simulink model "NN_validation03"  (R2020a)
settings: Solver=ode45  StartTime=0.0  StopTime=2000  RelTol=1e-3  EnableMultiTasking=on
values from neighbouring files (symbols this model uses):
  Ts = 0.2    [init_model.m]
libraries: neural x26

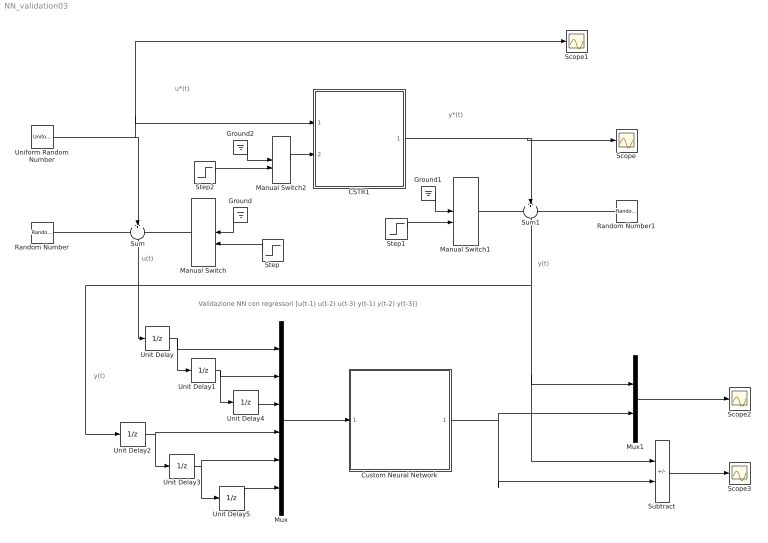
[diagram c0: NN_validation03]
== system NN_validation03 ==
  note: u(t)
  note: u*(t)
  note: y(t)
  note: y*(t)
  note: Validazione NN con regressori [u(t-1) u(t-2) u(t-3) y(t-1) y(t-2) y(t-3)]
  note: y(t)
  CSTR1 : Subsystem
  Custom Neural Network : Subsystem
      mask help: Custom Neural Network
  Ground : Ground
  Ground1 : Ground
  Ground2 : Ground
  Manual Switch : ManualSwitch  CurrentSetting=0
  Manual Switch1 : ManualSwitch
  Manual Switch2 : ManualSwitch
  Mux : Mux  Inputs=6
  Mux1 : Mux  Inputs=2
  Random Number : RandomNumber  Variance=0.0001  Seed=1  SampleTime=Ts
  Random Number1 : RandomNumber  Variance=0.0005  Seed=2  SampleTime=Ts
  Scope{,1..3} (4 alike) : Scope
  Step : Step  Time=1000  After=10  SampleTime=0
  Step1 : Step  Time=1000  After=10  SampleTime=0
  Step2 : Step  Time=1000  SampleTime=0
  Subtract : Sum  Inputs=+-
  Sum : Sum  Inputs=+++  SaturateOnIntegerOverflow=on
  Sum1 : Sum  Inputs=+++  SaturateOnIntegerOverflow=on
  Uniform Random Number : UniformRandomNumber  Minimum=0  Maximum=4  SampleTime=20
  Unit Delay{,1..5} (6 alike) : UnitDelay  SampleTime=Ts  HasFrameUpgradeWarning=on
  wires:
  Uniform Random Number/1 -> CSTR1/1(w), Scope1/1, Sum/2
  Random Number/1 -> Sum/1
  Manual Switch/1 -> Sum/3
  Sum/1 -> Unit Delay/1
  Ground/1 -> Manual Switch/1
  Step/1 -> Manual Switch/2
  Ground1/1 -> Manual Switch1/1
  Step1/1 -> Manual Switch1/2
  CSTR1/1(Cb) -> Scope/1, Sum1/2
  Manual Switch1/1 -> Sum1/1
  Random Number1/1 -> Sum1/3
  Unit Delay/1 -> Mux/1, Unit Delay1/1
  Unit Delay2/1 -> Unit Delay3/1, Mux/4
  Step2/1 -> Manual Switch2/2
  Manual Switch2/1 -> CSTR1/2(f)
  Ground2/1 -> Manual Switch2/1
  Unit Delay1/1 -> Mux/2, Unit Delay4/1
  Unit Delay4/1 -> Mux/3
  Unit Delay5/1 -> Mux/6
  Unit Delay3/1 -> Mux/5, Unit Delay5/1
  Mux/1 -> Custom Neural Network/1(Input)
  Subtract/1 -> Scope3/1
  Mux1/1 -> Scope2/1
  Sum1/1 -> Subtract/1, Mux1/1, Unit Delay2/1
  Custom Neural Network/1(Output) -> Subtract/2, Mux1/2

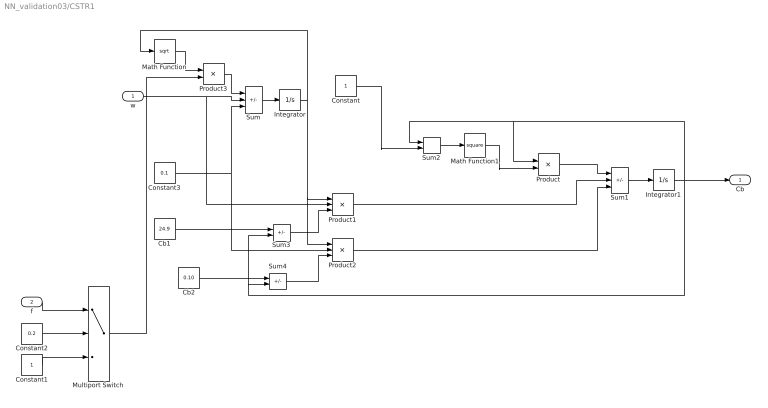
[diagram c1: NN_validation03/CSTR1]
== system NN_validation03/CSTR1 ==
  w : Inport
  f : Inport  Port=2
  Cb1 : Constant  Value=24.9
  Cb2 : Constant  Value=0.10
  Constant : Constant
  Constant1 : Constant
  Constant2 : Constant  Value=0.2
  Constant3 : Constant  Value=0.1
  Integrator : Integrator  InitialCondition=30  LimitOutput=on  LowerSaturationLimit=1
  Integrator1 : Integrator  InitialCondition=22
  Math Function : Math  Operator=sqrt
  Math Function1 : Math  Operator=square
  Multiport Switch : MultiPortSwitch  DataPortOrder=Zero-based contiguous  Inputs=2  zeroidx=on
  Product : Product  Inputs=*/  SaturateOnIntegerOverflow=on
  Product1 : Product  Inputs=/**  SaturateOnIntegerOverflow=on
  Product2 : Product  Inputs=/**  SaturateOnIntegerOverflow=on
  Product3 : Product
  Sum : Sum  Inputs=-++  SaturateOnIntegerOverflow=on
  Sum1 : Sum  Inputs=-++  SaturateOnIntegerOverflow=on
  Sum2 : Sum  SaturateOnIntegerOverflow=on
  Sum3 : Sum  Inputs=+-  SaturateOnIntegerOverflow=on
  Sum4 : Sum  Inputs=+-  SaturateOnIntegerOverflow=on
  Cb : Outport
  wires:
  Sum/1 -> Integrator/1
  Product3/1 -> Sum/1
  Math Function/1 -> Product3/1
  Integrator/1 -> Math Function/1, Product1/1, Product2/1
  Sum3/1 -> Product1/3
  Sum4/1 -> Product2/3
  Sum2/1 -> Math Function1/1
  Sum1/1 -> Integrator1/1
  Math Function1/1 -> Product/2
  Product/1 -> Sum1/1
  Product1/1 -> Sum1/2
  Product2/1 -> Sum1/3
  w/1 -> Sum/2, Product1/2
  Constant3/1 -> Product2/2, Sum/3
  Integrator1/1 -> Sum3/2, Sum4/2, Sum2/1, Product/1, Cb/1
  Constant1/1 -> Multiport Switch/3
  f/1 -> Multiport Switch/1
  Constant2/1 -> Multiport Switch/2
  Cb2/1 -> Sum4/1
  Cb1/1 -> Sum3/1
  Constant/1 -> Sum2/2
  Multiport Switch/1 -> Product3/2

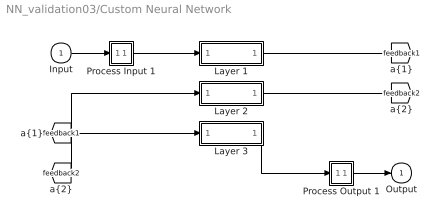
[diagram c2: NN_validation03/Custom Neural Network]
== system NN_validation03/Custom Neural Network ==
  Input : Inport  PortDimensions=6  SampleTime=0.2
  Layer 1 : Subsystem
  Layer 2 : Subsystem
  Layer 3 : Subsystem
  Process Input 1 : Subsystem
  Process Output 1 : Subsystem
  Output : Outport  InitialOutput=0
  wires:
  Input/1 -> Process Input 1/1(x)
  Process Output 1/1(y) -> Output/1
  Process Input 1/1(p) -> Layer 1/1("p{1}")
  Layer 1/1("a{1}") -> [feedback1]
  [feedback1] -> Layer 2/1("a{1} ")
  Layer 2/1("a{2}") -> [feedback2]
  [feedback2] -> Layer 3/1("a{2} ")
  Layer 3/1("a{3}") -> Process Output 1/1(a)

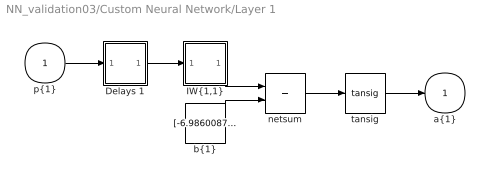
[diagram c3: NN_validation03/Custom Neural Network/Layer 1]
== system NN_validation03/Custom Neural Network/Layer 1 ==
  "p{1}" : Inport  PortDimensions=6  SampleTime=0.2
  Delays 1 : Subsystem
  "IW{1,1}" : Subsystem
  "b{1}" : Constant  Value=[-6.9860087142336624310701154172420501708984375;-1.3825822154357074733610488692647777497768402099609375;1.414744489111007030857081190333701670169830322265625;1.4343419531810190914455915844882838428020477294921875;0.364071132160834254332115733632235787808895111083984375;-0.2427588004599351700907305939836078323423862457275390625;-1.3732031975720901950666075208573602139949798583984375]
  netsum : Sum  Inputs=2  InputSameDT=on  SaturateOnIntegerOverflow=on
  tansig : neural/Transfer Functions/tansig
  "a{1}" : Outport  InitialOutput=[0;0;0;0;0;0;0]
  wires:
  "p{1}"/1 -> Delays 1/1("p{1}")
  Delays 1/1("pd{1,1}") -> "IW{1,1}"/1("pd{1,1}")
  "IW{1,1}"/1("iz{1,1}") -> netsum/1
  "b{1}"/1 -> netsum/2
  netsum/1 -> tansig/1
  tansig/1 -> "a{1}"/1

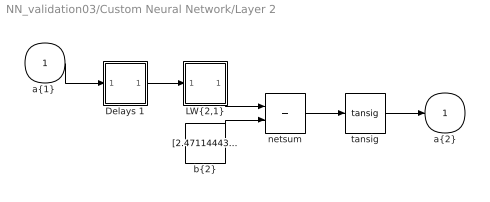
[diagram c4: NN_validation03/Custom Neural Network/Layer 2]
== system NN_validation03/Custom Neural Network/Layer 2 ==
  "a{1} " : Inport  PortDimensions=7  SampleTime=0.2
  Delays 1 : Subsystem
  "LW{2,1}" : Subsystem
  "b{2}" : Constant  Value=[2.471144434973719938852809718810021877288818359375;2.563750047572993739919411382288672029972076416015625;1.6633879212355908716602925778715871274471282958984375;-0.94058786412804240573137803949066437780857086181640625;-0.10710243137428977766578697128352359868586063385009765625;0.10718094125826170548432259010951383970677852630615234375;0.036160654709730725986371879798753070645034313201904296875;-0.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
  netsum : Sum  Inputs=2  InputSameDT=on  SaturateOnIntegerOverflow=on
  tansig : neural/Transfer Functions/tansig
  "a{2}" : Outport  InitialOutput=[0;0;0;0;0;0;0;0;0;0;0;0;0;0;0]
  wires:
  "a{1} "/1 -> Delays 1/1("p{2}")
  Delays 1/1("pd{2,1}") -> "LW{2,1}"/1("ad{2,1}")
  "LW{2,1}"/1("lz{2,1}") -> netsum/1
  "b{2}"/1 -> netsum/2
  netsum/1 -> tansig/1
  tansig/1 -> "a{2}"/1

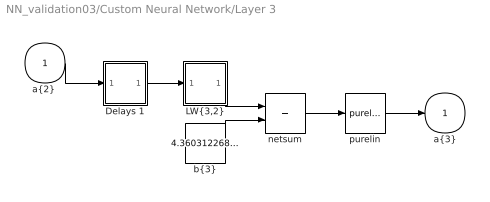
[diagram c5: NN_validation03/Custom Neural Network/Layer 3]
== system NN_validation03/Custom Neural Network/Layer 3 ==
  "a{2} " : Inport  PortDimensions=15  SampleTime=0.2
  Delays 1 : Subsystem
  "LW{3,2}" : Subsystem
  "b{3}" : Constant  Value=4.36031226847928454759539818041957914829254150390625
  netsum : Sum  Inputs=2  InputSameDT=on  SaturateOnIntegerOverflow=on
  purelin : neural/Transfer Functions/purelin
  "a{3}" : Outport  InitialOutput=0
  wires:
  "a{2} "/1 -> Delays 1/1("p{3}")
  Delays 1/1("pd{3,2}") -> "LW{3,2}"/1("ad{3,2}")
  "LW{3,2}"/1("lz{3,2}") -> netsum/1
  "b{3}"/1 -> netsum/2
  netsum/1 -> purelin/1
  purelin/1 -> "a{3}"/1

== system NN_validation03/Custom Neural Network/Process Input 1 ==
  x : Inport  PortDimensions=6  SampleTime=0.2
  p : Outport  PortDimensions=6  SampleTime=0.2
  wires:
  x/1 -> p/1

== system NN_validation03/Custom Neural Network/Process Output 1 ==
  a : Inport  PortDimensions=1  SampleTime=0.2
  y : Outport  PortDimensions=1  SampleTime=0.2
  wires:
  a/1 -> y/1

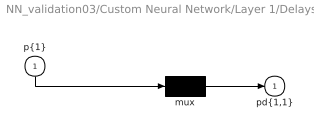
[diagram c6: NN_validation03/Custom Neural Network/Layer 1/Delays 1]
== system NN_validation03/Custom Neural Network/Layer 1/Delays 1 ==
  "p{1}" : Inport  PortDimensions=6  SampleTime=0.2
  mux : Mux  Inputs=1
  "pd{1,1}" : Outport
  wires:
  "p{1}"/1 -> mux/1
  mux/1 -> "pd{1,1}"/1

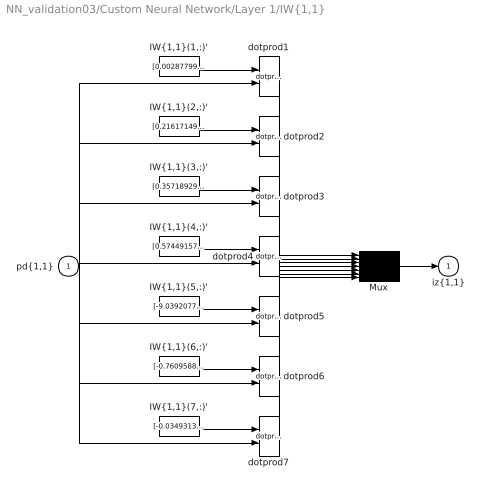
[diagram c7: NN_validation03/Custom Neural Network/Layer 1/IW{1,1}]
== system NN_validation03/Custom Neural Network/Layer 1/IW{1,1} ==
  "pd{1,1}" : Inport  PortDimensions=6  SampleTime=0.2
  "IW{1,1}(1,:)'" : Constant  Value=[0.0028779984139856201914853262024962532450444996356964111328125;0.0019664982693836491854655346145364092080853879451751708984375;-0.00147929606299945846752119660294511049869470298290252685546875;0.2128568022981623120148952921226737089455127716064453125;0.15321410908267463213405790156684815883636474609375;0.0028818070946959040146140296201338060200214385986328125]
  "IW{1,1}(2,:)'" : Constant  Value=[0.216171497179397709142989469910389743745326995849609375;-0.256379782057050531474118315600208006799221038818359375;1.216413369098526597866793963476084172725677490234375;1.2851285364890758788902758169570006430149078369140625;0.6513266071397028067480050594895146787166595458984375;0.89687545400963752939560436061583459377288818359375]
  "IW{1,1}(3,:)'" : Constant  Value=[0.357189298435218349769826318151899613440036773681640625;0.0770816338329727290812343198922462761402130126953125;0.1206306531016129446332030283883796073496341705322265625;0.1793601245096055618599706349414191208779811859130859375;-0.136347294813185138107058946843608282506465911865234375;0.534269401206287408712114483932964503765106201171875]
  "IW{1,1}(4,:)'" : Constant  Value=[0.57449157372489556561134804724133573472499847412109375;0.0535655250412447603292065423374879173934459686279296875;1.6300188103425783392452785847126506268978118896484375;-0.88950917467550916217788881112937815487384796142578125;-0.842863548106107085544635992846451699733734130859375;-0.71712381738132824349207794512039981782436370849609375]
  "IW{1,1}(5,:)'" : Constant  Value=[-9.039207732806421091709125903435051441192626953125;5.57292879519587902592547834501601755619049072265625;2.606658929916219502587182432762347161769866943359375;0.350236166318773911587669545042444951832294464111328125;1.842977695128436010918449028395116329193115234375;1.40701285377134244214403224759735167026519775390625]
  "IW{1,1}(6,:)'" : Constant  Value=[-0.760958801300770648623483793926425278186798095703125;-0.3305813588132300306909883147454820573329925537109375;0.9780848675967679373144392229733057320117950439453125;0.35816578911446528277195966438739560544490814208984375;0.215095185490126905580865468436968512833118438720703125;0.2030489209135220296520429883457836695015430450439453125]
  "IW{1,1}(7,:)'" : Constant  Value=[-0.034931350794894011624336371824028901755809783935546875;0.024790972801744672049384377032765769399702548980712890625;-0.2078553748513869148251131946381065063178539276123046875;-0.1817622112302082759693888647234416566789150238037109375;-0.2371104117750233164496620474892552010715007781982421875;-0.334586006731750262854774291554349474608898162841796875]
  Mux : Mux  Inputs=7
  dotprod{1..7} (7 alike) : neural/Weight Functions/dotprod
  "iz{1,1}" : Outport
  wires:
  "IW{1,1}(1,:)'"/1 -> dotprod1/1
  "pd{1,1}"/1 -> dotprod1/2, dotprod2/2, dotprod3/2, dotprod4/2, dotprod5/2, dotprod6/2, dotprod7/2
  dotprod1/1 -> Mux/1
  "IW{1,1}(2,:)'"/1 -> dotprod2/1
  dotprod2/1 -> Mux/2
  "IW{1,1}(3,:)'"/1 -> dotprod3/1
  dotprod3/1 -> Mux/3
  "IW{1,1}(4,:)'"/1 -> dotprod4/1
  dotprod4/1 -> Mux/4
  "IW{1,1}(5,:)'"/1 -> dotprod5/1
  dotprod5/1 -> Mux/5
  "IW{1,1}(6,:)'"/1 -> dotprod6/1
  dotprod6/1 -> Mux/6
  "IW{1,1}(7,:)'"/1 -> dotprod7/1
  dotprod7/1 -> Mux/7
  Mux/1 -> "iz{1,1}"/1

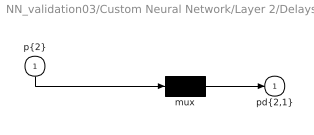
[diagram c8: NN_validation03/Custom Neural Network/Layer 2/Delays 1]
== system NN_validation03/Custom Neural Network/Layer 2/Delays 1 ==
  "p{2}" : Inport  PortDimensions=7  SampleTime=0.2
  mux : Mux  Inputs=1
  "pd{2,1}" : Outport
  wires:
  "p{2}"/1 -> mux/1
  mux/1 -> "pd{2,1}"/1

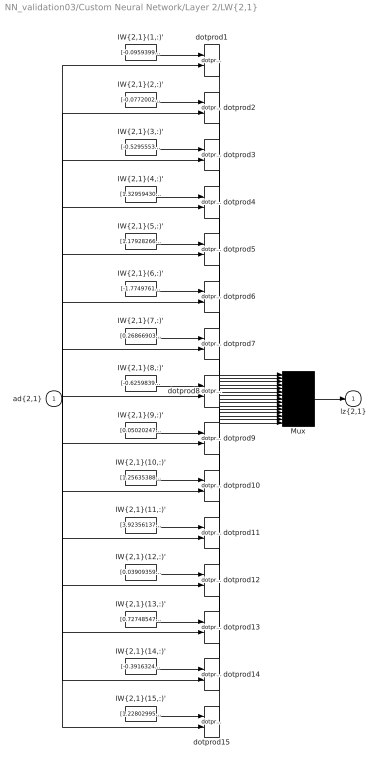
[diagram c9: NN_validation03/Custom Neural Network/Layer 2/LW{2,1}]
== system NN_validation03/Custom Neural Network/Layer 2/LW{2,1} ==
  "ad{2,1}" : Inport  PortDimensions=7  SampleTime=0.2
  "IW{2,1}(1,:)'" : Constant  Value=[-0.0959399622773860205615648055754718370735645294189453125;0.655443005093701458463328890502452850341796875;1.5326480917312477192382402790826745331287384033203125;0.273297613139449280250659057855955325067043304443359375;-0.494419526043682500127118828459060750901699066162109375;-0.442098376951397920020525589279714040458202362060546875;0.1081043964620367059392691544417175464332103729248046875]
  "IW{2,1}(10,:)'" : Constant  Value=[1.2563538867967849466111829315195791423320770263671875;0.2118795342555803984385676130841602571308612823486328125;0.97707874613680179010088977520354092121124267578125;-0.1634910230295236743813802604563534259796142578125;1.0634057917335013598858495242893695831298828125;0.0896381247422104454614100177423097193241119384765625;-1.449243030406923704589416956878267228603363037109375]
  "IW{2,1}(11,:)'" : Constant  Value=[3.92356137246147351760328092495910823345184326171875;0.346453038991754336262118840750190429389476776123046875;-0.8584902985731266422675389549112878739833831787109375;1.0809609548100904685696832530084066092967987060546875;-1.3582904381163312113045549267553724348545074462890625;-1.1984331101889231785406764174695126712322235107421875;0.64184409214700621770788302455912344157695770263671875]
  "IW{2,1}(12,:)'" : Constant  Value=[0.039093598208112589897922362069948576390743255615234375;0.5296252445861326929588130951742641627788543701171875;-0.407216201303665814581478343825438059866428375244140625;-0.93502189988382389262966398746357299387454986572265625;-1.4237866963899825645256669304217211902141571044921875;-0.79297346269186874678780441172420978546142578125;0.68312945034649630304812717440654523670673370361328125]
  "IW{2,1}(13,:)'" : Constant  Value=[0.7274854712775411513803192065097391605377197265625;-0.27024458002154327918020726428949274122714996337890625;0.8930885196710260931496350167435593903064727783203125;-0.393934283824690922859446118309278972446918487548828125;0.2197864491377925499904222306213341653347015380859375;-0.1984391574282319548050423918539308942854404449462890625;-1.764268177744925392147479215054772794246673583984375]
  "IW{2,1}(14,:)'" : Constant  Value=[-0.39163249261504484710627593813114799559116363525390625;-1.4803059639973021877068504181806929409503936767578125;-1.8821038698070602368517256763880141079425811767578125;-1.861443854278627352272224015905521810054779052734375;-1.0136653672223003841423860649229027330875396728515625;-1.8715655388637362221970761311240494251251220703125;0.4211240185482900688640484077041037380695343017578125]
  "IW{2,1}(15,:)'" : Constant  Value=[1.228029957202454891529441738384775817394256591796875;0.08383460798762738808154182379439589567482471466064453125;-0.1287360439631388686620994121767580509185791015625;-0.37687618205993944631160275093861855566501617431640625;1.3131633675176386244487503063282929360866546630859375;0.172747413149223316697344898784649558365345001220703125;-2.116416358688981258495687143295072019100189208984375]
  "IW{2,1}(2,:)'" : Constant  Value=[-0.07720026471078263174963041137743857689201831817626953125;-0.77642656336134752148581128494697622954845428466796875;-0.57078311752890387165138008640496991574764251708984375;-0.4459029626559087855497409691452048718929290771484375;-1.095937542092304539664837648160755634307861328125;0.46508991118670295339398990108747966587543487548828125;-0.5898791500863003189891742295003496110439300537109375]
  "IW{2,1}(3,:)'" : Constant  Value=[-0.52955539603377210777779282580013386905193328857421875;0.380695324827011349899663628093549050390720367431640625;1.490990668198310498127057144301943480968475341796875;0.8474388349253036967212437957641668617725372314453125;-0.321984096421327692372216233707149513065814971923828125;1.305526797567252206277998993755318224430084228515625;0.431354301728282873984454681703937239944934844970703125]
  "IW{2,1}(4,:)'" : Constant  Value=[1.3295943026519989604850024988991208374500274658203125;0.219168106709783538921243462027632631361484527587890625;-0.5937076469785085297559135142364539206027984619140625;2.24228703483500790838434113538824021816253662109375;-1.07502977103365626732056625769473612308502197265625;0.319354633821309075170091773543390445411205291748046875;0.951407207900434759295649200794287025928497314453125]
  "IW{2,1}(5,:)'" : Constant  Value=[1.1792826647421990049480200468678958714008331298828125;-1.3974250332944766483933562994934618473052978515625;0.052559963138450287167824370726521010510623455047607421875;0.7397855375498625374319772163289599120616912841796875;-0.933221159027975755151373959961347281932830810546875;-0.1605368854278859114259603302343748509883880615234375;0.77600580319520362504448485196917317807674407958984375]
  "IW{2,1}(6,:)'" : Constant  Value=[-1.7749761352877648779013952662353403866291046142578125;-0.705022215991891965103377515333704650402069091796875;-0.89106465072456264575606610378599725663661956787109375;-1.113940530555239671883782648365013301372528076171875;0.7018219326317403083947965569677762687206268310546875;0.52109634642023017203626977789099328219890594482421875;0.286050343846186827523325746369664557278156280517578125]
  "IW{2,1}(7,:)'" : Constant  Value=[0.268669035321024984863669260448659770190715789794921875;1.1047129548001723975403365329839289188385009765625;-0.394572828158680055654627949479618109762668609619140625;0.1351555578045449956814394454340799711644649505615234375;-0.2287877822372510194792738502655993215739727020263671875;-1.1642123682099525527888772558071650564670562744140625;1.3612638945307808935325510901748202741146087646484375]
  "IW{2,1}(8,:)'" : Constant  Value=[-0.62598392565256777420046319093671627342700958251953125;-0.7259163065658820190861888477229513227939605712890625;0.57230040912212754022903027362190186977386474609375;-0.96510061854865092367816714613582007586956024169921875;1.085885666211073186104840715415775775909423828125;0.7610160126531224644708117921254597604274749755859375;-1.4404073543343149932383084887987934052944183349609375]
  "IW{2,1}(9,:)'" : Constant  Value=[0.050202472949302807958549266231784713454544544219970703125;-2.252858402387201142147432619822211563587188720703125;-1.1641044986401525296315639934618957340717315673828125;0.193586999184280850183625943827792070806026458740234375;-0.050994778472113498624107563728102832101285457611083984375;-0.217491782693102153611874882699339650571346282958984375;0.74418604183696557274885208244086243212223052978515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
  Mux : Mux  Inputs=15
  dotprod{1..15} (15 alike) : neural/Weight Functions/dotprod
  "lz{2,1}" : Outport
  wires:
  "IW{2,1}(1,:)'"/1 -> dotprod1/1
  "ad{2,1}"/1 -> dotprod1/2, dotprod2/2, dotprod3/2, dotprod4/2, dotprod5/2, dotprod6/2, dotprod7/2, dotprod8/2, dotprod9/2, dotprod10/2, dotprod11/2, dotprod12/2, dotprod13/2, dotprod14/2, dotprod15/2
  dotprod1/1 -> Mux/1
  "IW{2,1}(2,:)'"/1 -> dotprod2/1
  dotprod2/1 -> Mux/2
  "IW{2,1}(3,:)'"/1 -> dotprod3/1
  dotprod3/1 -> Mux/3
  "IW{2,1}(4,:)'"/1 -> dotprod4/1
  dotprod4/1 -> Mux/4
  "IW{2,1}(5,:)'"/1 -> dotprod5/1
  dotprod5/1 -> Mux/5
  "IW{2,1}(6,:)'"/1 -> dotprod6/1
  dotprod6/1 -> Mux/6
  "IW{2,1}(7,:)'"/1 -> dotprod7/1
  dotprod7/1 -> Mux/7
  "IW{2,1}(8,:)'"/1 -> dotprod8/1
  dotprod8/1 -> Mux/8
  "IW{2,1}(9,:)'"/1 -> dotprod9/1
  dotprod9/1 -> Mux/9
  "IW{2,1}(10,:)'"/1 -> dotprod10/1
  dotprod10/1 -> Mux/10
  "IW{2,1}(11,:)'"/1 -> dotprod11/1
  dotprod11/1 -> Mux/11
  "IW{2,1}(12,:)'"/1 -> dotprod12/1
  dotprod12/1 -> Mux/12
  "IW{2,1}(13,:)'"/1 -> dotprod13/1
  dotprod13/1 -> Mux/13
  "IW{2,1}(14,:)'"/1 -> dotprod14/1
  dotprod14/1 -> Mux/14
  "IW{2,1}(15,:)'"/1 -> dotprod15/1
  dotprod15/1 -> Mux/15
  Mux/1 -> "lz{2,1}"/1

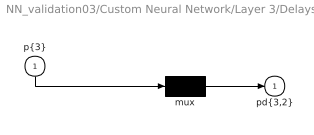
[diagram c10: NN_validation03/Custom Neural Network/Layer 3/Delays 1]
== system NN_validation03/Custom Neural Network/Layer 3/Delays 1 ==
  "p{3}" : Inport  PortDimensions=15  SampleTime=0.2
  mux : Mux  Inputs=1
  "pd{3,2}" : Outport
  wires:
  "p{3}"/1 -> mux/1
  mux/1 -> "pd{3,2}"/1

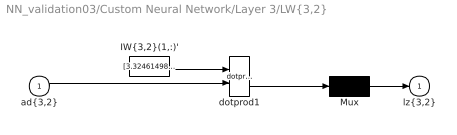
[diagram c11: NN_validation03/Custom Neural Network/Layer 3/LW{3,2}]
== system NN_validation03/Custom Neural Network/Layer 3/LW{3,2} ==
  "ad{3,2}" : Inport  PortDimensions=15  SampleTime=0.2
  "IW{3,2}(1,:)'" : Constant  Value=[3.32461498832466961772524882690049707889556884765625;3.737291852541816172816879770834930241107940673828125;0.55047621192276474655358242671354673802852630615234375;-1.5669689820374481659115417642169632017612457275390625;0.49511657157464927792034359299577772617340087890625;-1.8049088206470316197993497553397901356220245361328125;-1.206520046280243008141042082570493221282958984375;1.11734065969948459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
  Mux : Mux  Inputs=1
  dotprod1 : neural/Weight Functions/dotprod
  "lz{3,2}" : Outport
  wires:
  "IW{3,2}(1,:)'"/1 -> dotprod1/1
  "ad{3,2}"/1 -> dotprod1/2
  dotprod1/1 -> Mux/1
  Mux/1 -> "lz{3,2}"/1
